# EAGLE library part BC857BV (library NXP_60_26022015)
PNP double transistor in a SOT666 plastic package. NPN complement: BC847BV. AAL Eindhoven MK
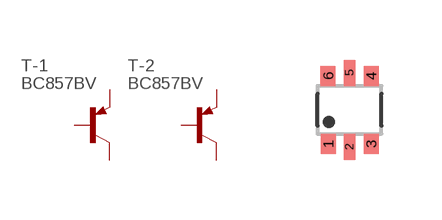
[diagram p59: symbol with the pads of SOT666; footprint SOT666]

Designator prefix T; gates -1=PNP -2=PNP

## BC857BV  [SOT666]
1  -1:E  pas
2  -1:B  pas
3  -2:C  pas
4  -2:E  pas
5  -2:B  pas
6  -1:C  pas

## Footprint SOT666 (pad centres in mm)
SOT 666 Reflow soldering foorprint Source: Philips - BAS70_1PS7XSB70_SER_8.pdf
smd 0.375 x 0.5: 1 -0.537,-0.85; 3 0.538,-0.85; 4 0.538,0.85; 6 -0.538,0.85
smd 0.3 x 0.65: 2 0,-0.925; 5 0,0.925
